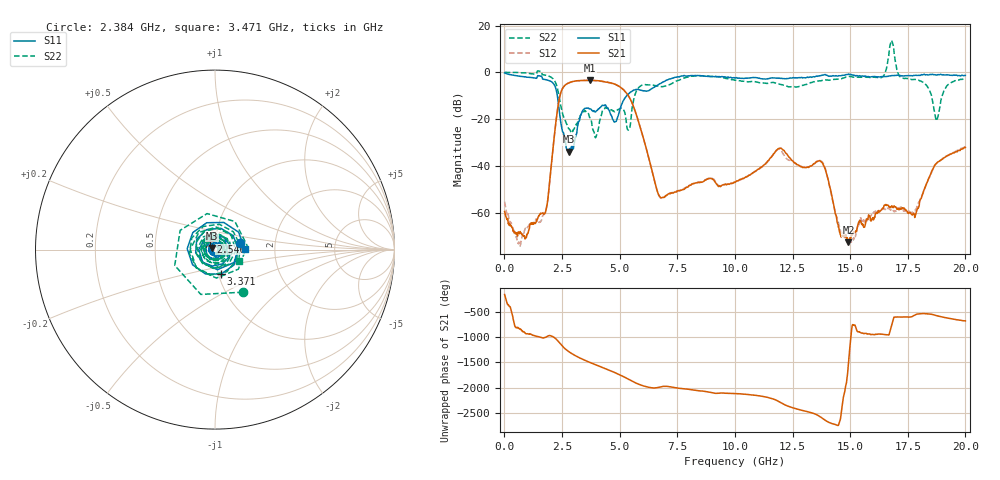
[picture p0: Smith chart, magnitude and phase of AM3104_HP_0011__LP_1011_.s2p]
!Created with skrf (http://scikit-rf.org).
# Hz S RI R 50.0
!freq ReS11 ImS11 ReS21 ImS21 ReS12 ImS12 ReS22 ImS22
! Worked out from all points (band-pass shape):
!   1601 points, 10 MHz to 20 GHz, reference 50 ohm
!   highest |S21| = -3.41 dB at 3.696 GHz (marker M1); lowest = -72.7 dB at 14.93 GHz (marker M2)
!   |S21| within 3 dB of the highest: 2.555 GHz to 5.035 GHz (2.48 GHz wide, 65.3 % of centre)
!   lowest |S11| = -34.0 dB at 2.796 GHz (marker M3), VSWR 1.04, Z = 48.3 + j0.941 ohm
!   |S11| at or under -10 dB: 2.298 GHz to 5.304 GHz (3.006 GHz wide, 79.1 % of centre)
!   |S22| runs from -28.0 to 13.6 dB; largest |S21 - S12| = 0.054
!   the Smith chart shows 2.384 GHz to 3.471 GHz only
!   S11 on the Smith chart (normalised r, x): 2.384 GHz: 1.32, +0.11; 2.546 GHz: 0.95, +0.09; 3.371 GHz: 1.03, -0.29; 3.471 GHz: 1.40, +0.01
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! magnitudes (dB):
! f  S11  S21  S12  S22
! 10 MHz  -0.3  -59.6  -55.4  0.0
! 647.2 MHz  -1.7  -68.7  -73.1  -0.2
! 1.634 GHz  -2.2  -60.3  -62.4  -0.7
! 2.384 GHz  -16.8  -11.3  -11.3  -10.9
! 2.546 GHz  -25.7  -6.5  -6.6  -18.4
! 2.796 GHz  -34.0  -4.5  -4.5  -24.1
! 3.346 GHz  -17.6  -3.5  -3.6  -17.5
! 3.371 GHz  -17.0  -3.5  -3.6  -16.9
! 3.471 GHz  -15.5  -3.5  -3.5  -16.7
! 3.696 GHz  -15.7  -3.4  -3.5  -19.3
! 5.395 GHz  -9.2  -10.3  -10.3  -24.7
! 5.807 GHz  -7.3  -20.7  -20.7  -6.8
! 6.682 GHz  -5.3  -52.2  -52.3  -6.0
! 10.01 GHz  -2.5  -47.1  -47.1  -3.4
! 11.93 GHz  -2.5  -32.5  -32.8  -5.1
! 13.34 GHz  -2.1  -39.9  -39.9  -4.4
! 13.84 GHz  -1.2  -39.7  -39.2  -3.5
! 14.93 GHz  -0.8  -72.7  -72.9  -1.8
! 16.68 GHz  -1.6  -57.4  -58.4  7.2
! 17.79 GHz  -1.4  -61.0  -59.3  -3.0
! 18.75 GHz  -1.2  -38.9  -38.8  -20.8
! 20 GHz  -1.3  -32.2  -31.9  -2.7
